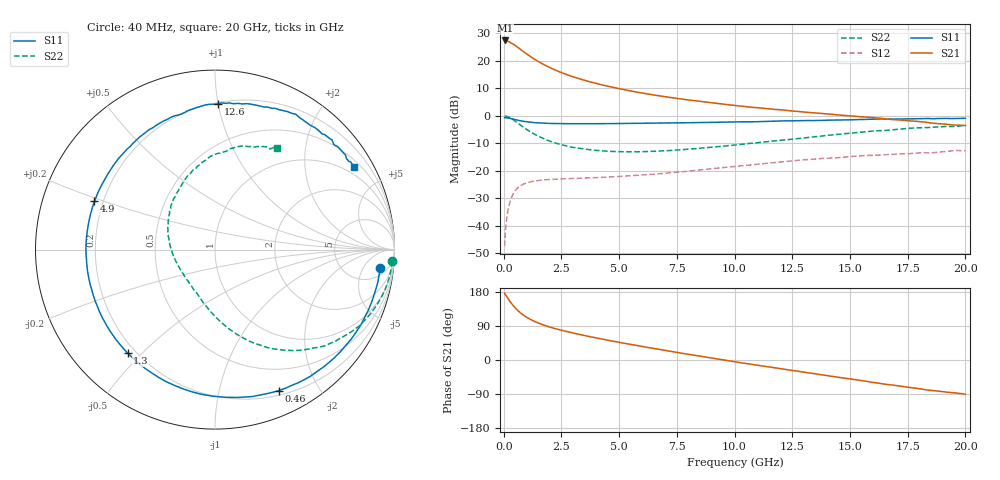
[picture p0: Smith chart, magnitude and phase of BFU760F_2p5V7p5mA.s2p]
! Filename:  P:\Prog\Test\Noise\ATS_data\Testdata_Net\Split files Spar\BFU760F_2W_C1_Bias2_2.5V_5mA_30mA_D.s2p
! Date/Time: Mon 06/Feb/2012 15:08:00
! BFU760_2W_C1_Bias2_2.5V_5mA_30mA_R.s2p
! MDIF S-parameter v. bias file
! BFU760_2W_C1_2.5V_5mA_30mA
! Date/time Fri Mar 18 11:16:19 2011
! VAR V_out= 2.5000
! VAR I_out= 7.4950
! VAR V_in= 0.7650
! VAR I_in= 0.0201
! Device data file deembeded for feedlines and parallel
! Original file: \Split files Spar\BFU760_2W_C1_Bias2_2.5V_5mA_30mA_R.s2p
! Feed-files: PR003V01_101208_Feed1.s2p, PR003V01_101208_Feed2.s2p
! Parallel-file: PR003V01_101208_Par.s2p
# MHz S MA R 50
!  Freq-MHz  S11-mag  S11-arg  S21-mag  S21-arg  S12-mag  S12-arg  S22-mag  S22-arg
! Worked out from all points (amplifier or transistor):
!   167 points, 40 MHz to 20 GHz, reference 50 ohm
!   highest |S21| = 27.4 dB at 50 MHz (marker M1)
!   |S21| within 3 dB of that: start of sweep to 685.5 MHz
!   unconditionally stable (mu >= 1): 5.559 GHz to 12.72 GHz
!   at 550 MHz: K = 0.10, MSG = 26.0 dB, |S12| = -26.7 dB
!   at 4.2 GHz: K = 0.81, MSG = 16.9 dB, |S12| = -22.4 dB
!   at 20 GHz: K = 0.80, MSG = 4.6 dB, |S12| = -12.6 dB
!   S11 on the Smith chart (normalised r, x): 40 MHz: 9, -12; 460 MHz: 0.25, -1.52; 1.3 GHz: 0.17, -0.45; 4.9 GHz: 0.17, +0.19; 12.6 GHz: 0.21, +1.00; 20 GHz: 0.72, +3.51
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40  0.9265 -6.2  23.38 176.1  0.004286 79.8  0.9897 -3.8
50  0.9267 -7.8  23.38 174.6  0.004952 79.9  0.9883 -4.8
140  0.9187 -21.5  22.88 166.4  0.01474 77.1  0.9729 -13.4
240  0.9034 -36.4  22.09 157.2  0.02445 70.1  0.9371 -22.4
340  0.8856 -50.1  20.81 149.0  0.0329 63.1  0.8878 -31.0
460  0.8621 -65.6  19.49 140.1  0.04132 55.8  0.8226 -39.8
600  0.8337 -81.2  17.68 131.1  0.04863 48.5  0.7434 -48.8
700  0.8171 -90.6  16.38 125.7  0.05264 44.2  0.691 -54.4
850  0.7957 -103.2  14.67 118.5  0.05735 38.8  0.6235 -61.5
1050  0.7727 -116.8  12.78 110.7  0.06151 33.4  0.5454 -69.3
1300  0.7544 -130.2  10.89 102.8  0.06501 28.5  0.472 -77.2
1650  0.7381 -144.2  8.922 94.0  0.06792 23.7  0.3982 -86.3
2100  0.7259 -157.5  7.179 85.0  0.07005 19.8  0.3353 -95.8
2700  0.7202 -170.6  5.667 75.5  0.07199 16.9  0.2832 -106.6
3400  0.7188 177.8  4.548 65.9  0.07382 15.1  0.2528 -117.8
4900  0.7234 158.2  3.176 47.7  0.0786 14.2  0.2241 -140.6
6800  0.7365 138.5  2.287 27.3  0.08893 14.2  0.2302 -166.8
10200  0.7766 108.5  1.514 -6.4  0.1224 8.1  0.3019 150.0
12600  0.8125 88.7  1.212 -28.6  0.153 -2.0  0.3799 124.4
13400  0.8191 82.8  1.135 -35.6  0.1633 -6.9  0.4118 116.0
16800  0.8732 55.9  0.858 -65.8  0.1988 -27.6  0.5525 83.3
20000  0.9012 30.7  0.6672 -90.4  0.2337 -50.0  0.6645 58.8
